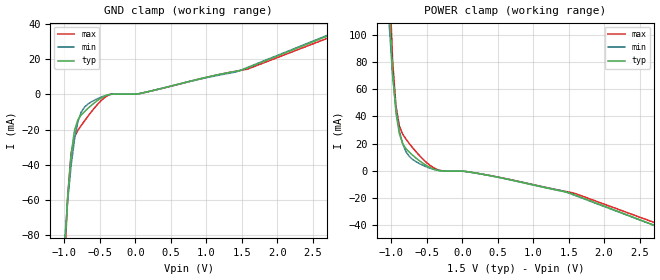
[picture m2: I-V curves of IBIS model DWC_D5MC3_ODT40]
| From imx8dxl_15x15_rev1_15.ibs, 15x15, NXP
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[Model] DWC_D5MC3_ODT40
Model_type   Input
Polarity   Non-Inverting
Enable   Active-High
C_comp   1.505pF   1.492pF   1.544pF
C_comp_power_clamp   572.866fF   450.742fF   593.000fF
C_comp_gnd_clamp 969.219fF   907.572fF   1.040pF
Vinh = 875.000mV
Vinl = 625.000mV
[Model Spec]
D_overshoot_ampl_h 0.4 NA   NA
D_overshoot_ampl_l 0.4 NA   NA
D_overshoot_area_l 100.000p NA   NA
D_overshoot_area_h 100.000p NA   NA
[Receiver Thresholds]
Vth = 750.000mV
Vth_min = 735.000mV
Vth_max = 765.000mV
Vinh_ac = 125.000mV
Vinh_dc = 100.000mV
Vinl_ac = -125.000mV
Vinl_dc = -100.000mV
Tslew_ac = 5.000ns
Threshold_sensitivity = 0.5
Reference_supply Power_clamp_ref
[Temperature Range]   25.000   125.000   -40.000
[Voltage Range]   1.500V   1.425V   1.575V
[GND Clamp Reference]   0.00V   0.00V   0.00V
[C Comp Corner]
| variable   typ   min   max
C_comp 1.544pF   1.492pF   1.505pF
C_comp_pullup 572.866fF   450.742fF   593.000fF
C_comp_pulldown 969.219fF   1.040pF   907.572fF
[POWER Clamp Reference]   1.500V   1.425V   1.575V
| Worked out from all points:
|   GND clamp passes 1 mA (typ) near -0.44 V on its own axis
|   POWER clamp passes 1 mA (typ) near -0.38 V on its own axis
[GND Clamp]
-1.48V    -900.7mA   -635.4mA   -1.159A
-1.002V   -92.53mA   -86.05mA   -99.8mA
-954.5mV  -58.56mA   -60.68mA   -58.3mA
-906.8mV  -34.65mA   -40.81mA   -33.68mA
-859.1mV  -20.55mA   -25.8mA    -24.19mA
-811.4mV  -14.45mA   -15.66mA   -20.49mA
-763.6mV  -11.67mA   -9.981mA   -17.66mA
-668.2mV  -7.88mA    -5.45mA    -12.36mA
-334.1mV  130.9uA    138.4uA    332.2uA
47.73mV   424.6uA    422uA      407.6uA
1.432V    13.35mA    13.02mA    13.37mA
2.959V    37.37mA    37.82mA    35.96mA
[Power Clamp]
-1.459V   1.013A     697.9mA    1.336A
-1.03V    121.7mA    107.1mA    143.9mA
-981.8mV  71.63mA    70.44mA    80.57mA
-934.1mV  42.53mA    45.25mA    47.45mA
-886.4mV  27.3mA     29.27mA    32.99mA
-838.6mV  19.9mA     19.53mA    26.86mA
-790.9mV  16.14mA    13.81mA    23.14mA
-647.7mV  9.241mA    6.646mA    13.81mA
-313.6mV  62.47uA    194uA      352.7uA
163.6mV   -1.37mA    -1.376mA   -1.33mA
1.405V    -14.93mA   -14.59mA   -14.59mA
2.979V    -45.38mA   -45.44mA   -43.07mA
